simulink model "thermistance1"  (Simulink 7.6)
settings: Solver=ode14x  SolverMode=SingleTasking  StartTime=0.0  StopTime=10.0  FixedStep=0.001  MaxStep=1e-6  RelTol=1e-3
InitFcn:
  | R=10;
  | Vcc=5;
StopFcn:
  | clc
libraries: fl_lib x13, nesl_utility x4, elec_lib x2

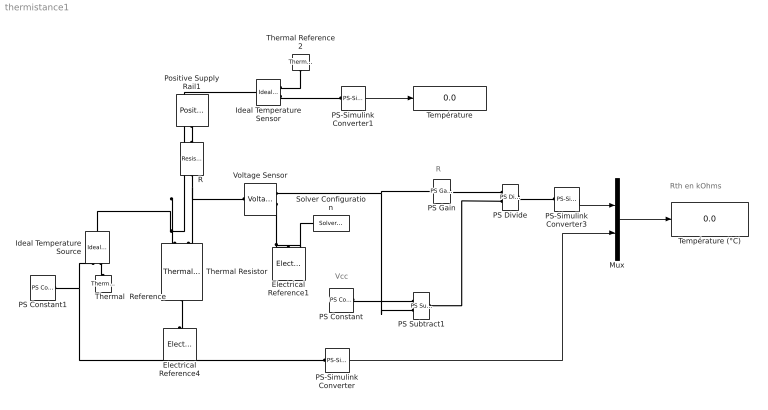
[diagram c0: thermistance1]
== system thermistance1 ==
  note: Rth en kOhms
  note: R
  note: Vcc
  Electrical Reference1 : fl_lib/Electrical/Electrical Elements/Electrical Reference  DialogController=NetworkEngine.DynNeDlgSource  SystemSampleTime=-1  i_Log=off  LocalVarNames=|i  LocalVarDescs=|i  LocalVarLogging=0
  Electrical Reference4 : fl_lib/Electrical/Electrical Elements/Electrical Reference  DialogController=NetworkEngine.DynNeDlgSource  SystemSampleTime=-1  i_Log=off  LocalVarNames=|i  LocalVarDescs=|i  LocalVarLogging=0
  Ideal Temperature Sensor : fl_lib/Thermal/Thermal Sensors/Ideal Temperature Sensor  DialogController=NetworkEngine.DynNeDlgSource  SystemSampleTime=-1  Qs_Log=off  Ts_Log=off  LocalVarNames=|Qs|Ts  LocalVarDescs=|Qs|Ts  LocalVarLogging=[0 0]
  Ideal Temperature Source : fl_lib/Thermal/Thermal Sources/Ideal Temperature Source  DialogController=NetworkEngine.DynNeDlgSource  SystemSampleTime=-1  Q_Log=off  T_Log=off  LocalVarNames=|Q|T  LocalVarDescs=|Q|T  LocalVarLogging=[0 0]
  Mux : Mux  Inputs=2
  PS Constant : fl_lib/Physical Signals/Sources/PS Constant  DialogController=NetworkEngine.DynNeDlgSource  SystemSampleTime=-1  constant=Vcc  LocalVarLogging=[]
  PS Constant1 : fl_lib/Physical Signals/Sources/PS Constant  DialogController=NetworkEngine.DynNeDlgSource  SystemSampleTime=-1  constant=50  LocalVarLogging=[]
  PS Divide : fl_lib/Physical Signals/Functions/PS Divide  DialogController=NetworkEngine.DynNeDlgSource  SystemSampleTime=-1  LocalVarLogging=[]
  PS Gain : fl_lib/Physical Signals/Functions/PS Gain  DialogController=NetworkEngine.DynNeDlgSource  SystemSampleTime=-1  gain=R  LocalVarLogging=[]
  PS Subtract1 : fl_lib/Physical Signals/Functions/PS Subtract  DialogController=NetworkEngine.DynNeDlgSource  SystemSampleTime=-1  LocalVarLogging=[]
  PS-Simulink Converter : nesl_utility/PS-Simulink Converter  DialogController=NetworkEngine.DynNeUtilDlgSource  SystemSampleTime=-1  PhysicalDomain=network_engine_domain  LeftPortType=input  RightPortType=output  SubClassName=ps_output  Unit=1  AffineConversion=off
  PS-Simulink Converter1 : nesl_utility/PS-Simulink Converter  DialogController=NetworkEngine.DynNeUtilDlgSource  SystemSampleTime=-1  PhysicalDomain=network_engine_domain  LeftPortType=input  RightPortType=output  SubClassName=ps_output  Unit=1  AffineConversion=off
  PS-Simulink Converter3 : nesl_utility/PS-Simulink Converter  DialogController=NetworkEngine.DynNeUtilDlgSource  SystemSampleTime=-1  PhysicalDomain=network_engine_domain  LeftPortType=input  RightPortType=output  SubClassName=ps_output  Unit=1  AffineConversion=off
  Positive Supply Rail1 : elec_lib/Sources/Positive Supply Rail  DialogController=NetworkEngine.DynNeDlgSource  SystemSampleTime=-1  v0=Vcc V  current_Log=off  voltage_Log=off  power_Log=off  LocalVarNames=|current|voltage|power  LocalVarDescs=|Current (A)|Voltage (V)|Power (W)  LocalVarLogging=[0 0 0]
  R : fl_lib/Electrical/Electrical Elements/Resistor  DialogController=NetworkEngine.DynNeDlgSource  SystemSampleTime=-1  R=R kOhm  i_Log=off  v_Log=off  LocalVarNames=|i|v  LocalVarDescs=|i|v  LocalVarLogging=[0 0]
  Solver Configuration : nesl_utility/Solver Configuration  DialogController=NetworkEngine.DynNeUtilDlgSource  SystemSampleTime=-1  PhysicalDomain=network_engine_domain  LeftPortType=input  RightPortType=generic  SubClassName=solver  Accelerate=off  Profile=off  ResidualTolerance=1e-9  MaxNonlinIter=12  MaxModeIter=2  DoFixedCost=off  UseLocalSampling=off  DoDC=on  LinearAlgebra=Full  LocalSolverSampleTime=.001  LocalSolverChoice=NE_BACKWARD_EULER_ADVANCER  UseLocalSolver=off
  Température : Display
  Température (°C) : Display
  Thermal  Reference : fl_lib/Thermal/Thermal Elements/Thermal Reference  DialogController=NetworkEngine.DynNeDlgSource  SystemSampleTime=-1  Q_Log=off  LocalVarNames=|Q  LocalVarDescs=|Q  LocalVarLogging=0
  Thermal Reference2 : fl_lib/Thermal/Thermal Elements/Thermal Reference  DialogController=NetworkEngine.DynNeDlgSource  SystemSampleTime=-1  Q_Log=off  LocalVarNames=|Q  LocalVarDescs=|Q  LocalVarLogging=0
  Thermal Resistor : elec_lib/Passive Devices/Thermal Resistor  DialogController=NetworkEngine.DynNeDlgSource  SystemSampleTime=-1  R0=47 kOhm  T0=25 C  alpha=5e-05 1/K  tc=10 s  K_d=0.001 W/K  init_temp=25 C  current_Log=off  voltage_Log=off  power_Log=off  temperature_Log=off  heat_flow_Log=off  LocalVarNames=|current|voltage|power|temperature|heat_flow  LocalVarDescs=|Resistor current (A)|Voltage across resistor (V)|Power (W)|Themistor temperature (K)|Heat flow (J/s)  LocalVarLogging=[0 0 0 0 0]
  Voltage Sensor : fl_lib/Electrical/Electrical Sensors/Voltage Sensor  DialogController=NetworkEngine.DynNeDlgSource  SystemSampleTime=-1  i1_Log=off  v1_Log=off  LocalVarNames=|i1|v1  LocalVarDescs=|i1|v1  LocalVarLogging=[0 0]
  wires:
  PS-Simulink Converter1/1 -> Température/1
  PS-Simulink Converter3/1 -> Mux/1
  PS-Simulink Converter/1 -> Mux/2
  Mux/1 -> Température (°C)/1
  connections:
  Thermal Resistor/LConn1 -- Ideal Temperature Source/LConn1 -- Ideal Temperature Sensor/LConn1
  R/LConn1 -- Thermal Resistor/LConn2 -- Voltage Sensor/LConn1
  Positive Supply Rail1/RConn1 -- R/RConn1
  Voltage Sensor/RConn2 -- Electrical Reference1/LConn1 -- Solver Configuration/RConn1
  Ideal Temperature Source/RConn2 -- Thermal  Reference/LConn1
  Ideal Temperature Sensor/RConn2 -- PS-Simulink Converter1/LConn1
  Thermal Reference2/LConn1 -- Ideal Temperature Sensor/RConn1
  Thermal Resistor/RConn1 -- Electrical Reference4/LConn1
  PS Gain/RConn1 -- PS Divide/LConn1
  PS Constant/RConn1 -- PS Subtract1/LConn1
  Voltage Sensor/RConn1 -- PS Subtract1/LConn2 -- PS Gain/LConn1
  PS Divide/RConn1 -- PS-Simulink Converter3/LConn1
  PS Constant1/RConn1 -- Ideal Temperature Source/RConn1 -- PS-Simulink Converter/LConn1
  PS Subtract1/RConn1 -- PS Divide/LConn2
